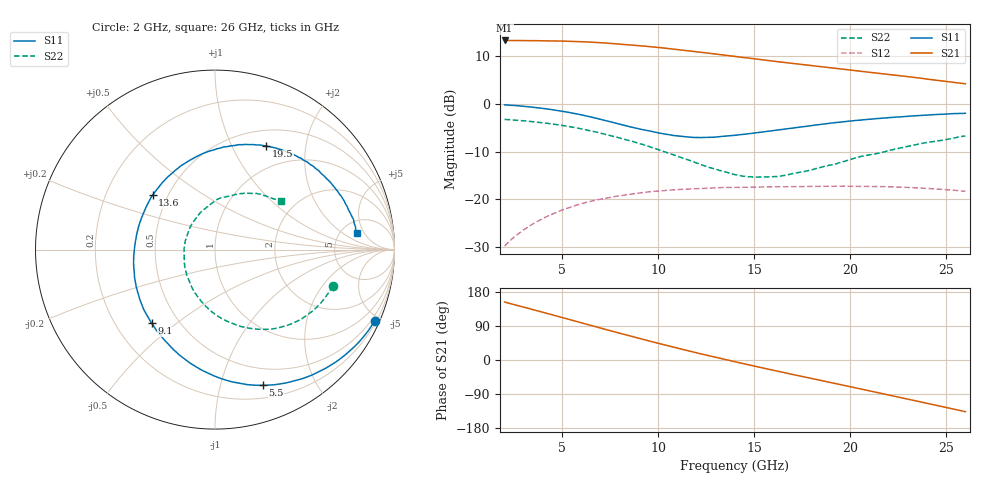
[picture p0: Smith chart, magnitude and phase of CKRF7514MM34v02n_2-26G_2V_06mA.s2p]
! CHUO DENSHI KOGYO Co.,Ltd.
! 22. July 2016
! CKRF7514MM34
! N-channel HJ-FET
! Vds = 2 V Id = 0 mA
# Hz S  MA  R 50
!	f	S11	S21	S12	S22
!	Hz	MAG	ANG	MAG	ANG	MAG	ANG	MAG	ANG
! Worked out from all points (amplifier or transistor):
!   241 points, 2 GHz to 26 GHz, reference 50 ohm
!   highest |S21| = 13.2 dB at 2 GHz (marker M1)
!   |S21| within 3 dB of that: start of sweep to 13.32 GHz
!   unconditionally stable (mu >= 1): 12.89 GHz to 19.97 GHz; 20.09274 GHz to 20.10131 GHz
!   at 6 GHz: K = 0.56, MSG = 16.9 dB, |S12| = -20.9 dB
!   at 14 GHz: K = 1.03, MAG = 12.7 dB, |S12| = -17.5 dB
!   at 26 GHz: K = 0.82, MSG = 11.2 dB, |S12| = -18.3 dB
!   lowest NFmin = 0.33 dB at 10 GHz
!   S11 on the Smith chart (normalised r, x): 2 GHz: 0.30, -4.68; 5.5 GHz: 0.32, -1.36; 9.1 GHz: 0.35, -0.41; 13.6 GHz: 0.41, +0.32; 19.5 GHz: 0.70, +1.37; 26 GHz: 6.99, +3.54
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2e9  0.9743 -24.0  4.589 152.8  0.0325 72.8  0.6865 -17.1
3e9  0.9399 -36.6  4.574 139.5  0.04823 64.9  0.664 -25.7
3.9e9  0.8982 -48.3  4.555 127.2  0.06192 57.3  0.637 -33.7
4.8e9  0.8475 -60.6  4.527 114.9  0.07479 49.8  0.6023 -42.1
5.5e9  0.8014 -70.6  4.488 105.1  0.08411 43.9  0.5711 -48.8
6e9  0.7653 -78.0  4.456 98.2  0.09028 39.8  0.5478 -53.8
6.7e9  0.7111 -88.9  4.382 88.4  0.09778 33.7  0.5101 -60.6
7.4e9  0.6569 -100.3  4.293 78.7  0.1045 28.1  0.4708 -67.7
8.1e9  0.6041 -112.4  4.188 69.2  0.1099 22.6  0.432 -74.9
9.1e9  0.5408 -130.7  4.032 55.9  0.1175 15.6  0.3798 -85.5
1e10  0.4965 -148.6  3.878 44.1  0.1228 8.9  0.3317 -96.5
1.08e10  0.4659 -165.2  3.729 33.9  0.1261 3.6  0.2924 -106.3
1.17e10  0.4468 176.1  3.556 22.6  0.1288 -2.2  0.2531 -119.2
1.26e10  0.4454 157.6  3.383 11.7  0.1308 -7.5  0.2187 -133.6
1.36e10  0.4611 139.0  3.195 -0.1  0.1338 -13.6  0.1915 -152.1
1.4e10  0.4686 131.9  3.122 -4.7  0.1336 -16.0  0.1819 -159.7
1.59e10  0.5219 103.9  2.808 -26.1  0.1356 -26.2  0.172 160.3
1.8e10  0.5915 78.9  2.503 -48.8  0.1369 -37.4  0.2046 120.7
1.95e10  0.6439 63.6  2.314 -65.0  0.1374 -46.0  0.2427 99.6
2.2e10  0.7163 40.8  2.024 -92.1  0.1357 -61.7  0.3219 70.6
2.39e10  0.761 23.5  1.823 -113.2  0.1307 -75.6  0.3913 52.7
2.6e10  0.7961 6.7  1.617 -136.4  0.1221 -91.6  0.4598 36.5
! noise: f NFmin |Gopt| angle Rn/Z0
1e+10  0.33  0.5  101.4  0.07
1.05e+10  0.35  0.476  109.9  0.06
1.1e+10  0.36  0.449  119.7  0.05
1.15e+10  0.39  0.419  128.9  0.05
1.2e+10  0.42  0.394  140.7  0.04
1.25e+10  0.42  0.372  152.9  0.04
1.3e+10  0.44  0.355  164.6  0.03
1.35e+10  0.47  0.349  178.3  0.03
1.4e+10  0.5  0.355  -168.7  0.03
1.5e+10  0.54  0.372  -146.6  0.04
